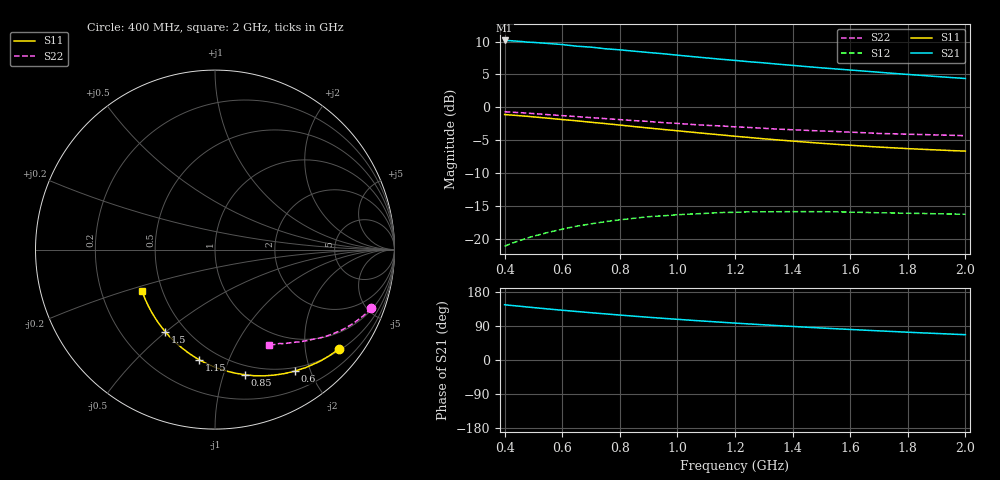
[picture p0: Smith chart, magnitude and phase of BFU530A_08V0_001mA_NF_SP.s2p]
! Filename:  P:\Prog\Test\Noise\ATS_data\Testdata_Net\06 Compressed Noise after Statistics\BFU530A_APG2013_33_A05_08p0V_001mA_SP_CM01_D.sf
! Date/Time: Tue 16/Apr/2013 15:10:55
! BFU530A_APG2013_33_A05_08p0V_1to25mA_NF_CM01_Bias1_R.sf
! Noise Parameter Data File
! BFU530A_APG2013_33_A05_08p0V_1to25mA_NF_CM01
! Date/time: Fri Apr 12 16:45:05 2013
! freq range =  0.4000 to  2.0000 GHz, 37 points
! bias range =  1.0050 to 25.0000 mA, 8 points
! bias supplies used: 1 1 0 0 0 0
! VAR bias_mode= 1  ! Specify V_out, I_out
! VAR bias_var = 1  ! Bias variable = I_out
! VAR V_out= 8.001000
! VAR I_out= 1.005000
! VAR V_in= 0.781800
! VAR I_in= 0.010001
! Device data file deembeded for feedlines and parallel
! Original file: \06 Compressed Noise after Statistics\BFU530A_APG2013_33_A05_08p0V_001mA_SP_CM01_R.sf
! Feed-files: PR017V01_150413_Feed1.s2p, PR017V01_150413_Feed2.s2p
! Parallel-file: PR017V01_150413_Par.s2p
# MHz S MA R 50
!  Freq-MHz  S11-mag  S11-arg  S21-mag  S21-arg  S12-mag  S12-arg  S22-mag  S22-arg
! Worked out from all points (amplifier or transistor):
!   37 points, 400 MHz to 2 GHz, reference 50 ohm
!   highest |S21| = 10.2 dB at 400 MHz (marker M1)
!   |S21| within 3 dB of that: start of sweep to 1.193 GHz
!   unconditionally stable (mu >= 1): nowhere
!   at 500 MHz: K = 0.23, MSG = 14.7 dB, |S12| = -19.5 dB
!   at 1.1 GHz: K = 0.48, MSG = 11.8 dB, |S12| = -16.1 dB
!   at 2 GHz: K = 0.88, MSG = 10.3 dB, |S12| = -16.2 dB
!   lowest NFmin = 0.51 dB at 420 MHz
!   S11 on the Smith chart (normalised r, x): 400 MHz: 0.54, -2.74; 600 MHz: 0.45, -1.77; 850 MHz: 0.41, -1.18; 1.15 GHz: 0.39, -0.78; 1.5 GHz: 0.39, -0.50; 2 GHz: 0.38, -0.23
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400  0.8844 -38.9  3.221 145.8  0.08882 65.5  0.9286 -20.5
420  0.877 -40.8  3.21 144.2  0.09244 64.4  0.9228 -21.4
440  0.8705 -42.6  3.186 142.7  0.09589 63.4  0.9173 -22.3
480  0.8564 -46.1  3.127 139.8  0.1025 61.3  0.9052 -24.0
500  0.8484 -47.9  3.115 138.3  0.1056 60.4  0.899 -24.8
550  0.8294 -52.4  3.058 134.8  0.1128 58.0  0.8826 -26.8
600  0.8099 -56.7  3 131.3  0.1195 55.8  0.8672 -28.7
650  0.7923 -60.6  2.915 128.1  0.1259 53.7  0.8533 -30.4
700  0.7725 -64.9  2.866 124.8  0.1311 51.7  0.8375 -32.2
750  0.7546 -68.8  2.786 121.7  0.1362 49.9  0.823 -33.8
800  0.7355 -72.8  2.735 118.6  0.1406 48.1  0.8088 -35.3
850  0.7165 -76.7  2.671 115.6  0.1446 46.4  0.7948 -36.8
950  0.6817 -84.2  2.555 110.0  0.1509 43.4  0.7681 -39.6
1050  0.6495 -91.3  2.432 104.8  0.1557 40.9  0.7437 -42.1
1150  0.6197 -98.3  2.322 99.8  0.1598 38.6  0.7247 -44.3
1200  0.6052 -101.7  2.274 97.4  0.1604 37.6  0.713 -45.5
1350  0.5673 -111.5  2.129 90.7  0.162 35.4  0.6854 -48.7
1500  0.5352 -121.1  1.998 84.4  0.162 33.8  0.6635 -51.6
1650  0.5088 -130.2  1.886 78.7  0.1602 33.3  0.6435 -54.5
1750  0.4943 -136.3  1.813 75.1  0.1586 33.5  0.6318 -56.2
1850  0.4819 -142.0  1.748 71.6  0.1573 33.9  0.624 -58.0
2000  0.4671 -150.7  1.659 66.8  0.155 35.6  0.6112 -60.7
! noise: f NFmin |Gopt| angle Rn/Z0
400  0.5286  0.6388  22.17  0.3518
460  0.5667  0.6279  25.99  0.366
600  0.618  0.6165  35.35  0.3354
800  0.637  0.5978  49.43  0.2628
1000  0.6976  0.5827  62.91  0.2415
1200  0.7495  0.61  74.3  0.2363
1400  0.7831  0.5899  89.37  0.1798
1600  0.8102  0.5587  101.7  0.1538
1800  0.6681  0.5562  117.4  0.1063
2000  0.8516  0.5529  132.6  0.0802
